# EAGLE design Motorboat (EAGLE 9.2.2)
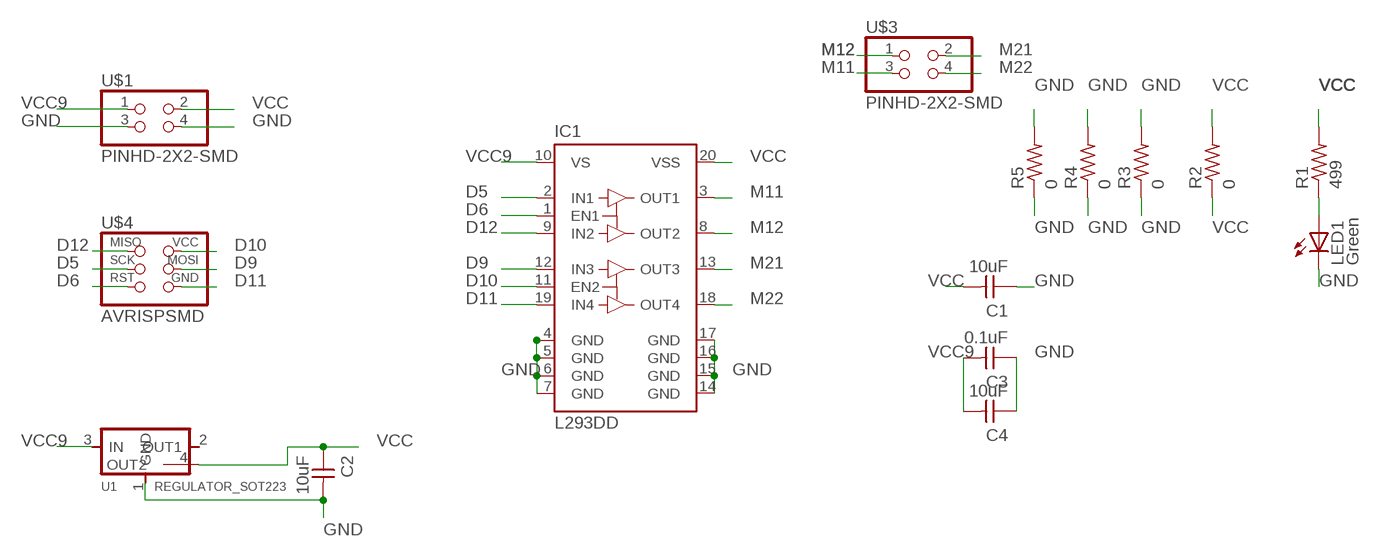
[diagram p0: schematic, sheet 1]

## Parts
C1  10uF  CAP-UNPOLARIZEDFAB  [C1206FAB]
C2  10uF  CAP-UNPOLARIZEDFAB  [C1206FAB]
C3  0.1uF  CAP-UNPOLARIZEDFAB  [C1206FAB]
C4  10uF  CAP-UNPOLARIZEDFAB  [C1206FAB]
IC1  L293DD  [SO20]
LED1  Green  LEDFAB1206  [LED1206FAB]
R1  499  RES-US1206FAB  [R1206FAB]
R2  0  RES-US1206FAB  [R1206FAB]
R3  0  RES-US1206FAB  [R1206FAB]
R4  0  RES-US1206FAB  [R1206FAB]
R5  0  RES-US1206FAB  [R1206FAB]
U1  REGULATOR_SOT223  [SOT223]
U$1  PINHD-2X2-SMD  [2X02SMD]
U$3  PINHD-2X2-SMD  [2X02SMD]
U$4  AVRISPSMD  [2X03SMD]

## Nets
D5: IC1.2(IN1) U$4.3(SCK)
D6: IC1.1(EN1) U$4.5(RST)
D9: IC1.12(IN3) U$4.4(MOSI)
D10: IC1.11(EN2) U$4.2(VCC)
D11: IC1.19(IN4) U$4.6(GND)
D12: IC1.9(IN2) U$4.1(MISO)
GND: C1.1 C2.2 C3.1 C4.1 IC1.4(GND) IC1.5(GND) IC1.6(GND) IC1.7(GND) IC1.14(GND) IC1.15(GND) IC1.16(GND) IC1.17(GND) LED1.2(C) R3.1 R3.2 R4.1 R4.2 R5.1 R5.2 U1.1(GND) U$1.3 U$1.4
M11: IC1.3(OUT1) U$3.3
M12: IC1.8(OUT2) U$3.1
M21: IC1.13(OUT3) U$3.2
M22: IC1.18(OUT4) U$3.4
N$2: LED1.1(A) R1.1
VCC: C1.2 C2.1 IC1.20(VSS) R1.2 R2.1 R2.2 U1.4(OUT2) U$1.2
VCC9: C3.2 C4.2 IC1.10(VS) U1.3(IN) U$1.1
Unconnected: U1.2(OUT1)

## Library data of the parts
C1-C4 = fab:CAP-UNPOLARIZED
IC1 = st-microelectronics:L293DD: PUSH-PULL FOUR CHANNEL DRIVER WITH DIODES Source: http://www.st.com/stonline/books/pdf/docs/1330.pdf; OC_FARNELL: unknown
LED1 = fab:LED: LED
R1-R5 = fab:RES-US: Resistor (US Symbol)
U1 = fab:REGULATOR_SOT223
U$1 U$3 = fab:PINHD-2X2-SMD
U$4 = fab:AVRISP

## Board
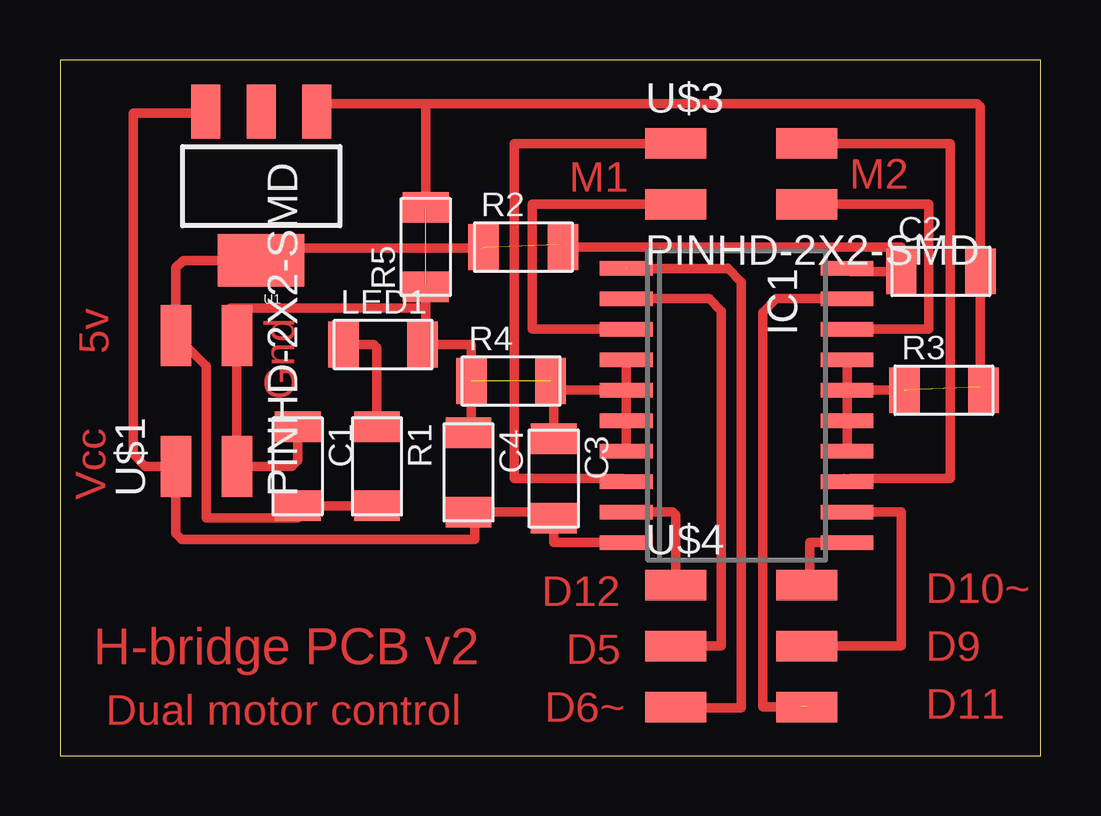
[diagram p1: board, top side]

Size 40.87 x 29.01 mm. Coordinates in mm from the lower left corner, seen from the top.
Outline: 0,0 40.87,0 40.87,29.01 0,29.01 0,0
Copper layers (1*16): Top 0.035mm / dielectric 1.5mm / Bottom 0.035mm
Design rules "default *": minimum track width 0.4mm, minimum drill 0.35mm, track to track 0.3mm, track to pad 0.3mm, pad to pad 0.3mm, via to via 0.3mm, smd to smd 0.3mm, copper to edge 40mil, drill to drill 6mil, minimum pad ring 10mil, minimum via ring 8mil, stop-mask expansion 4mil, vias tented up to drill 0mil, thermal gap 10mil

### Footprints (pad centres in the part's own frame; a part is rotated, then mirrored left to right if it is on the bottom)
C1206FAB = smd 1.27 x 1.905: 1 -1.651,0; 2 1.651,0
SO20 = smd 0.6 x 2.2: 1 -5.715,-4.6; 2 -4.445,-4.6; 3 -3.175,-4.6; 4 -1.905,-4.6; 5 -0.635,-4.6; 6 0.635,-4.6; 7 1.905,-4.6; 8 3.175,-4.6; 9 4.445,-4.6; 10 5.715,-4.6; 11 5.715,4.6; 12 4.445,4.6; 13 3.175,4.6; 14 1.905,4.6; 15 0.635,4.6; 16 -0.635,4.6; 17 -1.905,4.6; 18 -3.175,4.6; 19 -4.445,4.6; 20 -5.715,4.6
LED1206FAB = smd 1.27 x 1.905: 1 -1.651,0; 2 1.651,0
R1206FAB = smd 1.27 x 1.905: 1 -1.651,0; 2 1.651,0
SOT223 = smd 1.219 x 2.235: 1 -2.311,-3.099; 2 0,-3.099; 3 2.311,-3.099 | smd 3.6 x 2.2: 4 0,3.099
2X02SMD = smd 2.54 x 1.27: 1 -2.54,1.27; 2 2.92,1.27; 3 -2.54,-1.27; 4 2.92,-1.27
2X03SMD = smd 2.54 x 1.27: 1 -2.54,2.54; 2 2.92,2.54; 3 -2.54,0; 4 2.92,0; 5 -2.54,-2.54; 6 2.92,-2.54

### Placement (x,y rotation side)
C1  9.91,12.07 270 top
C2  36.7,20.19 0 top
C3  20.57,11.56 270 top
C4  17.02,11.81 270 top
IC1  28.19,14.61 270 top
LED1  13.46,17.14 0 top
R1  13.21,12.07 270 top
R2  19.3,21.21 0 top
R3  36.83,15.24 0 top
R4  18.8,15.62 0 top
R5  15.24,21.21 90 top
U1  8.38,23.75 180 top
U$1  6.1,14.61 90 top
U$3  28.19,24.26 0 top
U$4  28.19,4.57 0 top

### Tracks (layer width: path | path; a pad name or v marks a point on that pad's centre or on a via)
D5
  Top 0.4: IC1.2 27.05,19.05 27.56,18.54 27.56,4.57 U$4.3
D6  (1 unrouted)
  Top 0.4: U$4.5 25.69,2 28.39,2 28.39,19.75 27.81,20.32 27.8,20.31 23.61,20.31
D9
  Top 0.4: 32.67,10.03 IC1.12 35.05,10.16 35.05,4.57 U$4.4 31.5,4.95 32.1,4.95
D10
  Top 0.4: U$4.2 31.24,7.24 31.24,8.89 IC1.11
D11  (1 unrouted)
  Top 0.4: 32.41,19.05 IC1.19 29.84,19.05 29.27,18.48 29.27,2.03 30.86,2.03
D12
  Top 0.4: U$4.1 25.65,10.03 25.53,10.16 IC1.9
GND  (4 unrouted)
  Top 0.3: R4.1 17.02,15.49
  Top 0.4: IC1.4 IC1.5 | IC1.5 IC1.6 IC1.7 | IC1.17 IC1.16 | IC1.16 IC1.15 IC1.14 | IC1.16 35.31,15.24 | 38.61,15.11 R3.2 38.35,15.37 C2.2 38.35,27.05 38.23,27.18 15.24,27.18 | IC1.5 20.83,15.24 R4.2 20.57,15.49 C3.1 | C4.1 17.14,13.59 R4.1 17.14,17.14 LED1.2 15.24,17.27 15.24,18.67 | C1.1 9.91,12.32 9.65,12.07 U$1.3 7.37,17.14 | 7.37,17.14 U$1.4 | 15.24,27.18 11.02,27.18 U1.1 | 15.24,18.67 7.11,18.67 7.11,17.4 7.37,17.14 | R5.2 15.24,27.18 | 15.24,18.67 R5.1
M11
  Top 0.4: 26.42,22.99 U$3.3 19.68,22.99 19.68,17.78 IC1.3
M12
  Top 0.4: U$3.1 18.92,25.53 18.92,11.56 23.47,11.56 IC1.8
M21
  Top 0.4: 32.67,11.56 IC1.13 32.92,11.56 37.08,11.56 37.08,25.53 U$3.2
M22
  Top 0.4: U$3.4 36.19,22.99 36.19,17.78 34.42,17.78 33.02,17.78 IC1.18
N$2
  Top 0.4: LED1.1 13.08,17.14 13.21,17.02 R1.1
VCC  (2 unrouted)
  Top 0.3: 21.08,21.34 R2.2
  Top 0.4: IC1.20 32.92,20.19 34.92,20.19 | 20.83,21.34 R2.2 35.05,21.21 34.92,21.08 34.92,20.19 | 17.6,21.16 8.89,21.16 U1.4 5.13,20.65 4.83,20.34 U$1.2 6.1,16.25 6.1,9.91 9.91,9.91 C1.2 R1.2 | C2.1 34.92,20.19
VCC9
  Top 0.4: IC1.10 20.57,8.89 C3.2 20.32,10.16 C4.2 17.27,9.91 17.27,9.02 5.08,9.02 4.83,9.27 U$1.1 3.56,12.07 3.05,12.57 3.05,26.8 6.02,26.8 U1.3

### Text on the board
Top: M1 | M2 | 5v | Gnd | Vcc | D10~ | D12 | H-bridge PCB v2 | D5 | D9 | Dual motor control | D6~ | D11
